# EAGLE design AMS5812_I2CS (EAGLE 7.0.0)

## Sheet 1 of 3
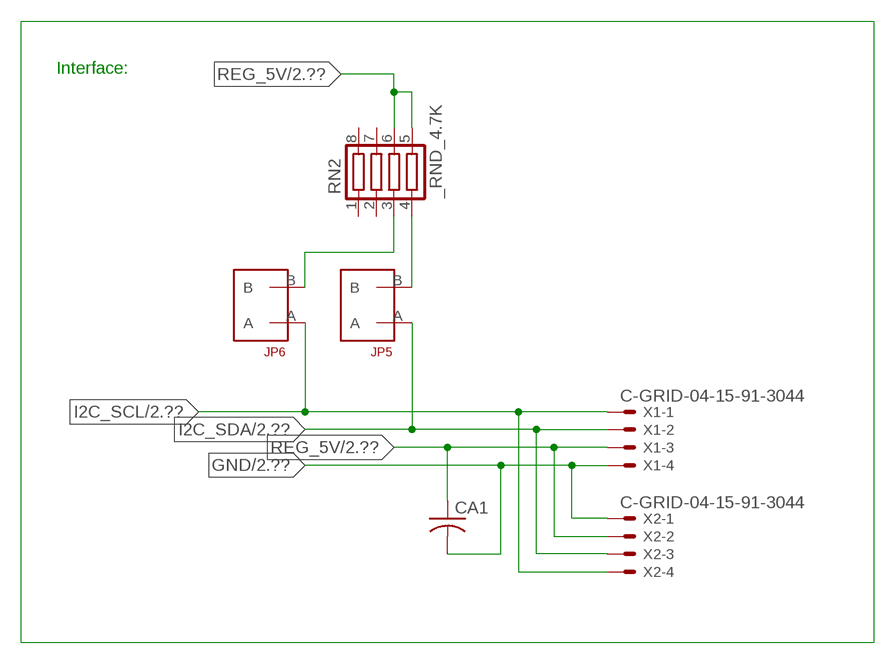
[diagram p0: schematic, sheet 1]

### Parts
CA1  CC1206KRX7R9BB104  [.1UF]
JP5  JUMPER_1X2_2MM  [JUMPER_1X2_2MM]
JP6  JUMPER_1X2_2MM  [JUMPER_1X2_2MM]
RN2  _RND_4.7K  [RND]
X1  C-GRID-04-15-91-3044  [15-91-04]
X2  C-GRID-04-15-91-3044  [15-91-04]

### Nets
GND: CA1.2 X1.4 X2.1 ; also sheet 2,3
I2C_SCL: JP6.A X1.1 X2.4 ; also sheet 2
I2C_SDA: JP5.A X1.2 X2.3 ; also sheet 2
N$1: JP6.B RN2.3
N$2: JP5.B RN2.4
REG_5V: CA1.1 RN2.5 RN2.6 X1.3 X2.2 ; also sheet 2,3
Unconnected: RN2.1 RN2.2 RN2.7 RN2.8

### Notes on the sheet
- Interface:

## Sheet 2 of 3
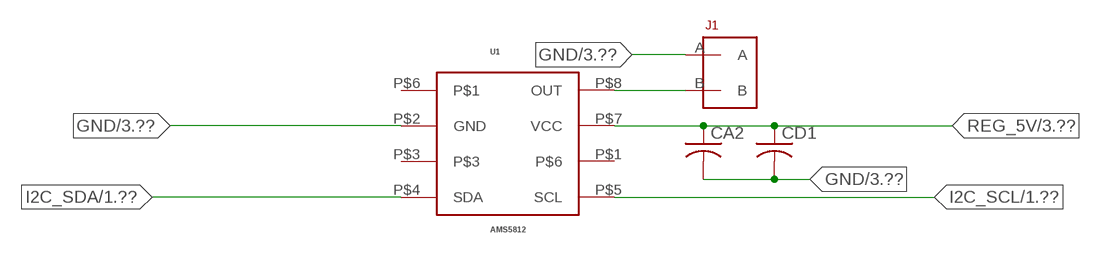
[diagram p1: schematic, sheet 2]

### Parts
CA2  _CA_.10UF_50VC1206K  [_CA_.1UF_50V]
CD1  _CD_10NF_50VC1206K  [_CD_10NF_50V]
J1  JUMPER_1X2_2MM  [JUMPER_1X2_2MM]
U1  AMS5812  [AMS5915]

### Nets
GND: CA2.2 CD1.2 J1.A U1.P$2(GND) ; also sheet 1,3
I2C_SCL: U1.P$5(SCL) ; also sheet 1
I2C_SDA: U1.P$4(SDA) ; also sheet 1
N$9: J1.B U1.P$8(OUT)
REG_5V: CA2.1 CD1.1 U1.P$7(VCC) ; also sheet 1,3
Unconnected: U1.P$1 U1.P$3 U1.P$6

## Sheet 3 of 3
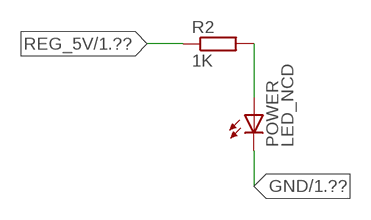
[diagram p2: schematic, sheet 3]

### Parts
POWER  LED_NCD  [CHIPLED_0603]
R2  1K  RESISTOR_SMT-0402  [R402]

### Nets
GND: POWER.C ; also sheet 1,2
N$3: POWER.A R2.2
REG_5V: R2.1 ; also sheet 1,2

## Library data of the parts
CA1 = NCD_ULTIMATE_LIBRARY:CC1206KRX7R9BB104: Capacitor CA .1uF 50V SMT C1206K CC1206KRX7R9BB104
CA2 = NCD_ULTIMATE_LIBRARY:_CA_.10UF_50V: Capacitor .1uF SMT
CD1 = NCD_ULTIMATE_LIBRARY:_CD_10NF_50V: Capacitor 10nF SMT
J1 JP5 JP6 = NCD_ULTIMATE_CONNECTORS:JUMPER_1X2_2MM
POWER = NCD_ULTIMATE_LIBRARY:LED_NCD: LED Digikey 754-1132-2-ND/APT2012SRCPRV
R2 = NCD_ULTIMATE_LIBRARY:RESISTOR_SMT: NCD Resistor
RN2 = NCD_ULTIMATE_LIBRARY:_RND_4.7K: Resistor Array RND SMT 4.7K x 4 Single Resistor Source: http://www.ctscorp.com/components/Datasheets/CTSChipArrayDs.pdf Digikey 742C083472JPTR-ND/742C083472JP; OC_FARNELL: unknown; OC_NEWARK: unknown
U1 = NCD_ULTIMATE_bhaskar:AMS5812
X1 X2 = NCD_ULTIMATE_CONNECTORS:C-GRID-04: CONNECTOR 4-Pos I2C wire to board 2.54 mm (0.100") pitch header Digikey WM1342-ND/0015912045; OC_FARNELL: unknown; OC_NEWARK: unknown

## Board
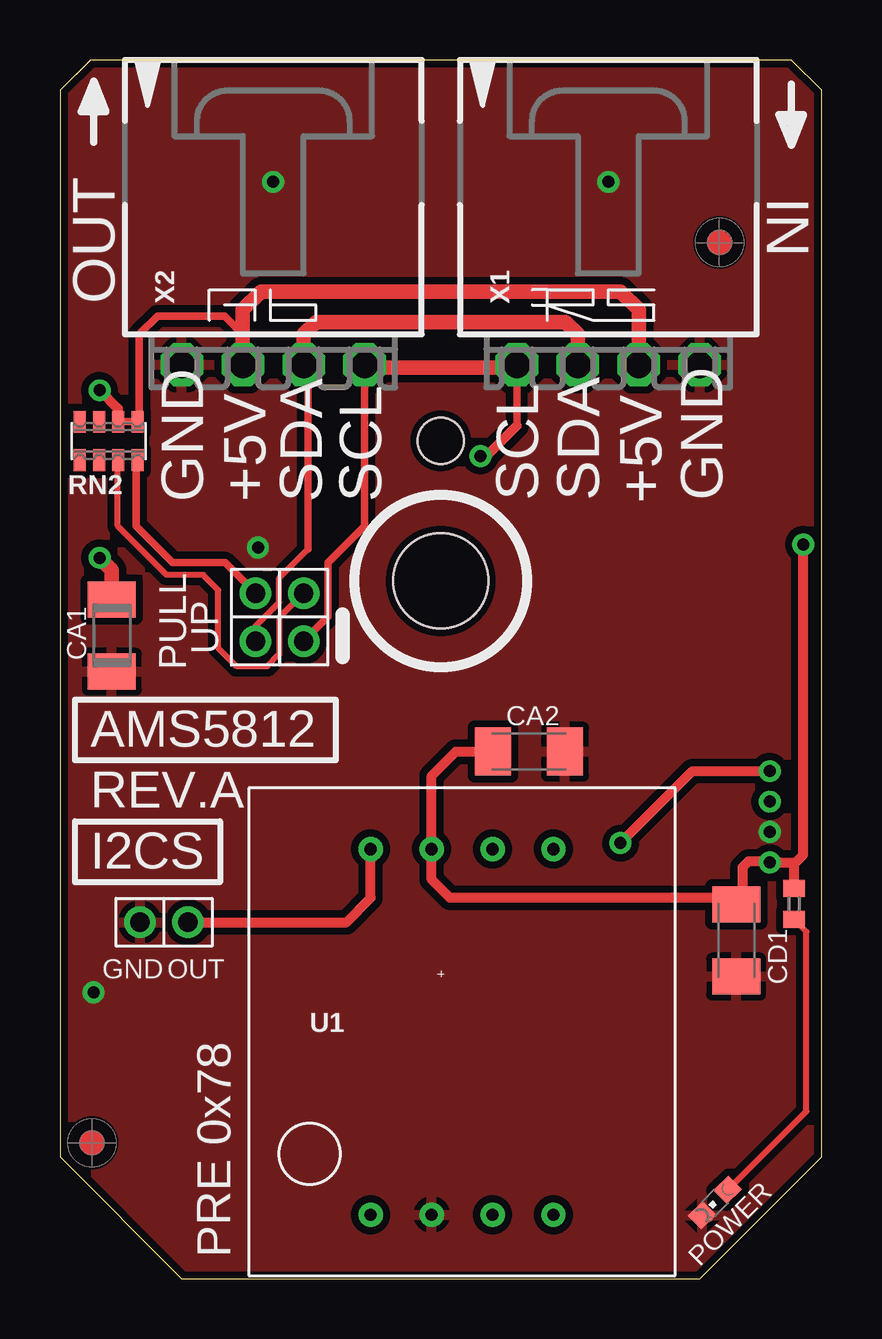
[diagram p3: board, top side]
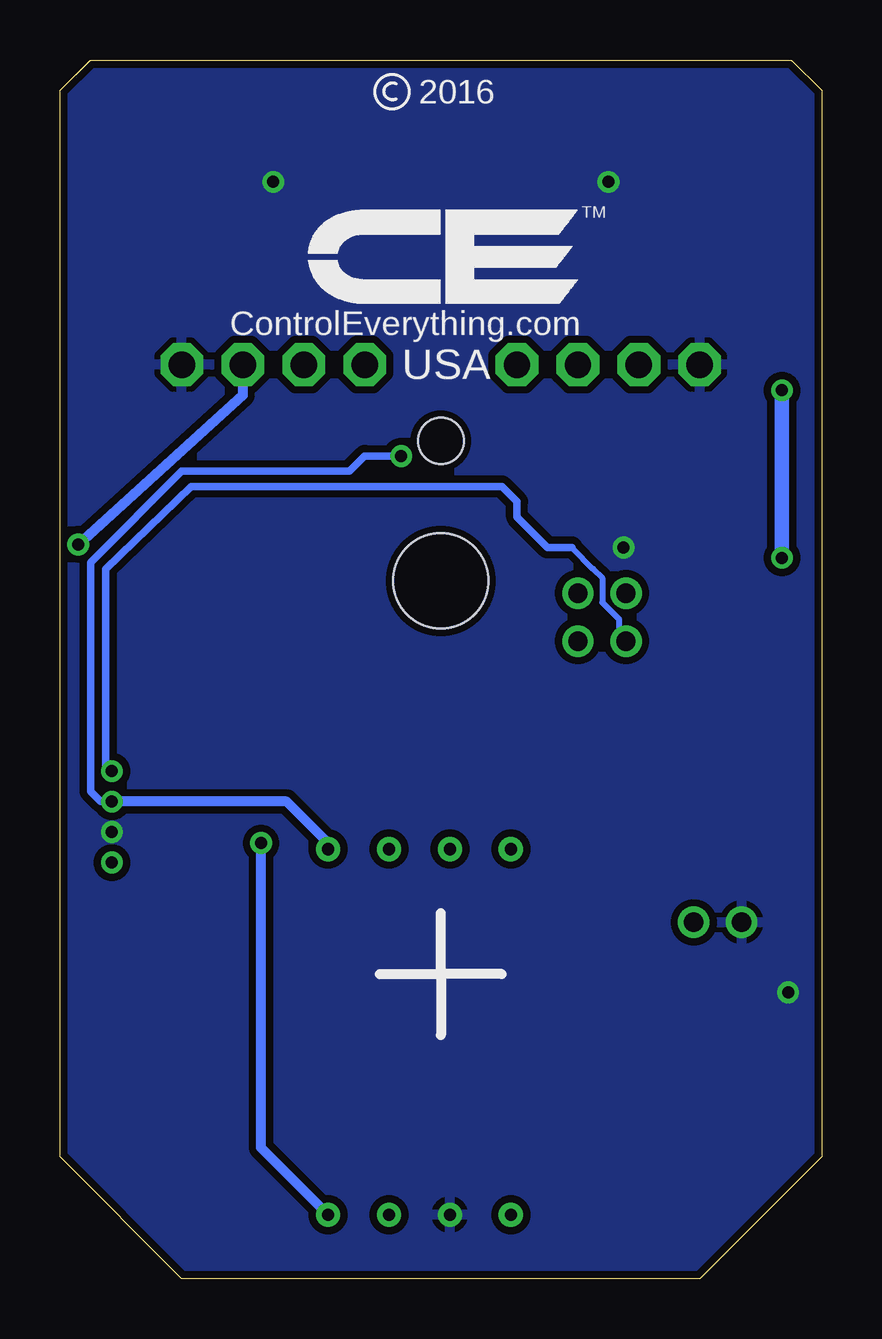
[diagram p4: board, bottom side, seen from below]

Size 31.75 x 50.8 mm. Coordinates in mm from the lower left corner, seen from the top.
Outline: 48 segments
Copper layers (1*16): Top 0.035mm / dielectric 1.5mm / Bottom 0.035mm
Design rules "default": minimum track width 5mil, minimum drill 24mil, track to track 5mil, track to pad 5mil, pad to pad 5mil, via to via 5mil, smd to smd 5mil, copper to edge 10mil, drill to drill 8mil, minimum pad ring 10mil, minimum via ring 8mil, stop-mask expansion 2mil, vias tented up to drill 0mil, thermal gap 10mil
Holes 3.96 mm at 15.88,29.08
Holes 1.91 mm at 15.88,34.92

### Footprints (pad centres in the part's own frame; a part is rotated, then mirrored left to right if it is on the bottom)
.1UF = smd 1.5 x 2: 1 -1.5,0; 2 1.5,0
_CA_.1UF_50V = smd 1.5 x 2: 1 -1.5,0; 2 1.5,0
_CD_10NF_50V = smd 1.5 x 2: 1 -1.5,0; 2 1.5,0
JUMPER_1X2_2MM = drill 0.8: A 0,2; B 0,0
CHIPLED_0603 = smd 0.8 x 0.876: A 0,-0.75; C 0,0.75
R402 = smd 0.7 x 0.9: 1 -0.65,0; 2 0.65,0
RND = smd 0.5 x 0.9: 1 -1.2,-0.8; 2 -0.4,-0.8; 3 0.4,-0.8; 4 1.2,-0.8; 5 1.2,0.8; 6 0.4,0.8; 7 -0.4,0.8; 8 -1.2,0.8
AMS5915 = drill 0.508: P$1 -2.54,-5.08; P$2 0,-5.08; P$3 2.54,-5.08; P$4 5.08,-5.08; P$5 5.08,10.16; P$6 2.54,10.16; P$7 0,10.16; P$8 -2.54,10.16
15-91-04 = drill 1.1 pad 1.778 octagon: 1 -3.81,-7.62; 2 -1.27,-7.62; 3 1.27,-7.62; 4 3.81,-7.62

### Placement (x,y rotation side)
CA1  2.16,26.81 270 top
CA2  19.56,21.97 0 top
CD1  28.19,14.1 270 top
J1  5.33,14.86 90 top
JP5  8.15,28.58 180 top
JP6  10.16,28.58 180 top
POWER  27.3,3.18 135 top
R2  30.61,15.62 270 top
RN2  2.03,34.92 0 top
U1  15.49,7.75 0 top
U$5  [VISION_REF10]  1.33,5.66 90 top
U$28  [VISION_REF10]  27.5,43.19 90 top
X1  22.86,45.72 0 top
X2  8.89,45.72 0 top

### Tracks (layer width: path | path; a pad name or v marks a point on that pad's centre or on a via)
GND  (via drill 0.5)
  other vias: 8.89,45.72 22.86,45.72 29.59,18.62 1.4,11.94 8.26,30.48
  pour Bottom (isolate 0.305): 4.45,-0.63 -0.63,4.45 -0.63,50.17 0.64,51.44 31.12,51.44 32.38,50.17 32.38,4.45 27.3,-0.63
  pour Top (isolate 0.305): 3.81,-1.27 -1.27,3.81 -1.27,50.8 0,52.07 31.75,52.07 33.02,50.8 33.02,3.81 27.94,-1.27
I2C_SCL  (via drill 0.5)
  Top 0.305: JP6.A 11.18,27.61 11.18,29.85 12.7,31.37 12.7,37.97 | 19.05,35.56 X1.1
  Top 0.406: X2.4 12.7,37.97 | 19.05,37.97 X1.1 | 19.05,35.56 17.78,34.29 v17.53,34.29
  Top 0.61: 12.7,37.97 19.05,37.97
  Bottom 0.305: v29.59,19.89 30.05,19.89 30.48,20.32 30.48,29.85 26.67,33.66 19.69,33.66 19.05,34.29 v17.53,34.29
  Bottom 0.406: U1.P$5 20.32,17.91 22.3,19.89 v29.59,19.89
I2C_SDA  (via drill 0.5)
  Top 0.254: JP5.A 8.15,27.2 9.14,28.19 9.14,29.21 10.35,30.42
  Top 0.305: 10.35,30.42 10.35,37.91 X2.3
  Top 0.406: v23.37,18.16 26.37,21.16 v29.59,21.16
  Top 0.61: X2.3 10.16,39.37 10.67,39.88 21.08,39.88 21.59,39.37 X1.2
  Bottom 0.254: 10.41,30.48 9.52,29.59 9.14,29.21 9.14,28.19 8.45,27.5 8.45,26.87 JP5.A
  Bottom 0.305: 10.41,30.48 11.43,30.48 12.7,31.75 12.7,32.39 13.34,33.02 26.29,33.02 29.85,29.59 29.85,21.41 v29.59,21.16
  Bottom 0.406: U1.P$4 23.37,5.46 v23.37,18.16
N$1
  Top 0.254: JP6.B | JP6.B 9.14,27.56 9.14,26.04 8.64,25.53 7.37,25.53 6.6,26.29 6.6,28.7 5.97,29.34 4.45,29.34 2.41,31.37 2.41,34.11 RN2.3
N$2
  Top 0.305: JP5.B 6.88,29.85 4.7,29.85 3.18,31.37 3.18,34.07 RN2.4
N$3
  Top 0.254: POWER.A 31.12,6.99 31.12,14.46 R2.2
N$9
  Top 0.406: J1.B 11.94,14.86 12.95,15.88 U1.P$8
REG_5V  (via drill 0.5)
  Top 0.305: 7.62,39.37 7.49,39.37 | RN2.6 RN2.5 3.3,35.8 3.3,39.37 4.06,40.13 6.86,40.13 7.62,39.37 | 7.62,40.39 7.62,39.37
  Top 0.406: 30.48,17.35 v29.59,17.35 29.54,17.4 28.7,17.4 28.45,17.15 28.45,15.37 | 30.48,17.35 30.67,17.35 30.99,17.67 v30.99,30.61 | v1.65,37.03 2.41,36.27 2.41,35.74 RN2.6 | CA2.1 16.51,21.97 15.49,20.96 U1.P$7 15.49,16.64 16.26,15.88 27.94,15.88 28.45,15.37 | 28.45,15.37 28.45,15.11 28.19,15.37 CD1.1 | R2.1 30.61,17.22 30.48,17.35
  Top 0.61: X1.3 24.13,38.23 24.13,40.39 23.37,41.15 8.38,41.15 7.62,40.39 X2.2 | CA1.1 2.16,29.54 v1.65,30.05
  Bottom 0.406: v30.99,30.61 24.13,36.83 24.13,37.47 24.16,38.08 24.13,38.23 X1.3
  Bottom 0.61: v1.65,30.05 v1.65,37.03

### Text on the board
tNames: IN | OUT | GND | +5V | SDA | SCL | SCL | SDA | +5V | GND | UP | PULL | AMS5812 | REV.A | I2CS | GND | OUT | PRE 0x78
bNames: 2016 | TM | ControlEverything.com | USA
